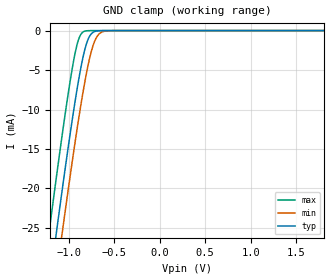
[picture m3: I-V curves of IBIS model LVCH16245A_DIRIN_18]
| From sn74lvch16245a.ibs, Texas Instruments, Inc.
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[Model]   LVCH16245A_DIRIN_18
Model_type  Input
Vinl=0.5775
Vinh=1.2675
| variable   typ   min   max
C_comp   2.70pF   2.13pF   3.31pF
[Temperature Range]   40   100   -40
| Ambient temperature   25   85   -40
[Voltage range]   1.8   1.65   1.95
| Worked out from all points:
|   GND clamp passes 1 mA (typ) near -0.78 V on its own axis
[GND Clamp]
| LVCH16245A_DIRIN_18
|   Voltage   I(typ)   I(min)   I(max)
-5V       -385.1mA   -389.7mA   -379.3mA
-1.21V    -32.27mA   -37.74mA   -25.26mA
-1.135V   -25.77mA   -31.24mA   -18.75mA
-1.075V   -20.67mA   -26.12mA   -13.69mA
-1.06V    -19.42mA   -24.86mA   -12.46mA
-960mV    -11.38mA   -16.66mA   -4.866mA
-885mV    -6.001mA   -10.91mA   -980.1uA
-830mV    -2.824mA   -7.089mA   -113.2uA
-780mV    -970.8uA   -4.107mA   -11.31uA
-715mV    -135.5uA   -1.404mA   -533.3nA
-650mV    -14.52uA   -292.8uA   -25.02nA
1.8V      3.325pA    5.318pA    3.026pA
